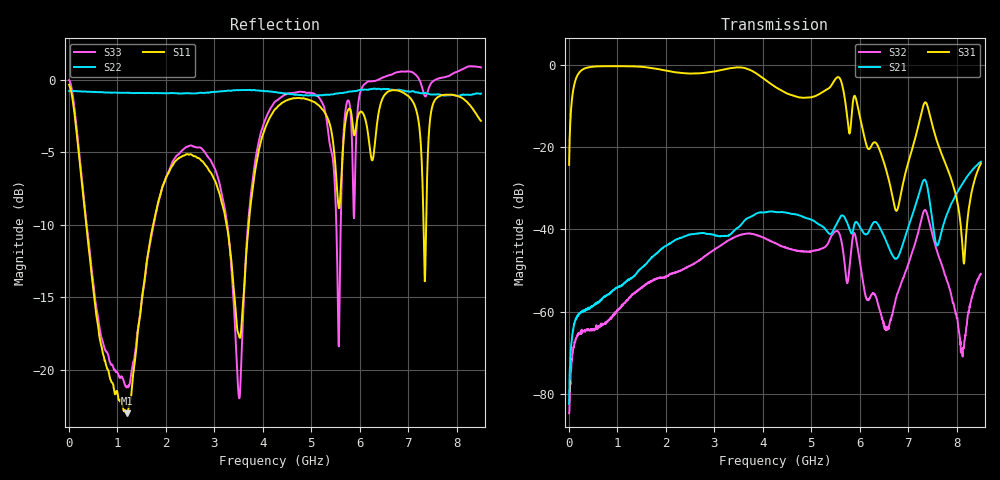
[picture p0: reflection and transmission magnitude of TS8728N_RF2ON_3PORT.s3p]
!Created with skrf (http://scikit-rf.org).
# GHz S RI R 50.0
!freq ReS11 ImS11 ReS12 ImS12 ReS13 ImS13
! ReS21 ImS21 ReS22 ImS22 ReS23 ImS23
! ReS31 ImS31 ReS32 ImS32 ReS33 ImS33
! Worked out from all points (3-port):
!   1601 points, 10 MHz to 8.5 GHz, reference 50 ohm
!   strongest paths, dB at 10 MHz, 2.132 GHz, 4.255 GHz, 6.378 GHz, 8.5 GHz:
!     S31: -24.3, -1.6, -5.3, -19.7, -23.9
!     S21: -82.4, -43.1, -35.7, -38.7, -23.5
!     S32: -84.8, -50.6, -43.2, -58.1, -50.8
!   lowest |S11| = -23.0 dB at 1.199 GHz (marker M1), VSWR 1.15, Z = 56.3 + j4.14 ohm
!   |S11| at or under -10 dB: 360.8 MHz to 1.743 GHz (1.382 GHz wide, 131 % of centre); 3.256 GHz to 3.713 GHz (457.1 MHz wide, 13.1 % of centre); 7.317 GHz to 7.37 GHz (53.06 MHz wide, 0.722 % of centre)
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0.01  -0.9574 0.0765  2.18e-07 5.95e-05  0.00533 0.0609
      -3.76e-07 7.56e-05  -0.9139 0.00519  1.82e-05 3.86e-05
      0.00534 0.0609  -3.14e-07 5.79e-05  -0.9938 0.0607
1.1986  0.0605 0.0366  -0.000192 0.00236  0.8757 -0.4203
        -0.000228 0.00233  -0.8239 0.3661  -0.00129 -0.000423
        0.8757 -0.4203  -0.0013 -0.000432  0.00413 0.0866
3.0664  -0.421 0.0578  0.00168 0.00821  0.2503 -0.815
        0.00169 0.00819  -0.4313 0.7994  -0.00195 0.0057
        0.2513 -0.816  -0.00197 0.00568  -0.3366 -0.3241
3.517431  -0.1272 -0.0248  -0.000868 0.0108  -0.0984 -0.9359
          -0.000896 0.0108  -0.3602 0.8472  0.00123 0.00842
          -0.0992 -0.9357  0.00125 0.00842  -0.0633 0.0482
4.255  -0.7491 -0.2531  0.00702 0.0148  -0.3616 -0.4092
       0.00702 0.0148  -0.2608 0.8681  0.00563 0.00393
       -0.362 -0.4091  0.00562 0.00398  0.2417 0.8042
6.1228  -0.4514 0.5666  0.00567 0.0066  -0.0944 0.0675
        0.0057 0.00663  0.3103 0.8706  0.00108 -0.00107
        -0.0943 0.0677  0.00108 -0.00108  0.0705 -0.9686
7.09915  -0.0259 0.8384  -0.0103 0.0119  0.0452 -0.0924
         -0.0103 0.0119  0.5313 0.7419  -0.000855 0.00556
         0.0453 -0.0925  -0.000882 0.00558  1.057 0.0407
7.385688  -0.3096 0.2905  0.0208 0.0284  -0.2534 -0.2192
          0.0208 0.0284  0.5815 0.6851  0.0158 0.00236
          -0.254 -0.2185  0.0157 0.00234  0.6808 0.5758
8.149788  0.5658 0.6433  -0.0164 0.0347  -0.000726 -0.00378
          -0.0164 0.0347  0.7102 0.5341  -0.000369 -0.000134
          -0.000715 -0.00377  -0.000338 -0.000164  -0.532 0.9562
8.5  0.7021 -0.1645  0.00633 0.0666  0.059 -0.0238
     0.00637 0.0665  0.7876 0.4256  -0.00168 0.00237
     0.0591 -0.024  -0.00164 0.00236  -1.051 0.3313
